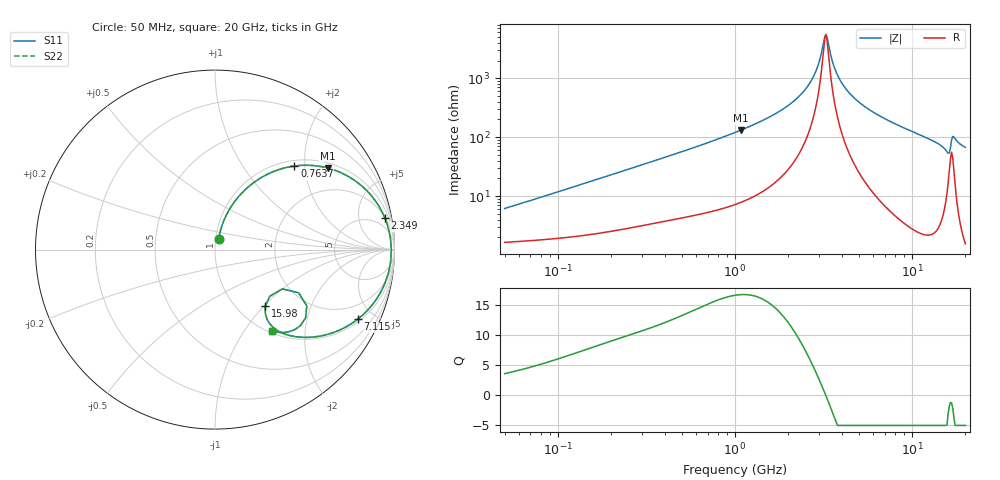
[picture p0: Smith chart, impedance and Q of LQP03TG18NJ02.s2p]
!Murata Part Number: LQP03TG18NJ02
!These Parameters are Measured in Series Mode Connection
!  o--[Z]--o
!Port1  Port2
!  o-------o
!Freq. Start=50[MHz] Stop=20[GHz], 401[Steps]
# Hz S RI R 50
!Freq.(Hz) S11(Real) S11(Imag) S21(Real) S21(Imag) S12(Real) S12(Imag) S22(Real) S22(Imag)
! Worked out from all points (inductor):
!   401 points, 50 MHz to 20 GHz, reference 50 ohm
!   read as one part in series: L = 18.8 nH near 51.52 MHz
!   highest Q = 16.8 at 1.078 GHz (marker M1), where L = 19.4 nH
!   self-resonance near 3.217 GHz
!   S11 on the Smith chart (normalised r, x): 50 MHz: 1.03, +0.12; 763.7 MHz: 1.11, +1.77; 2.349 GHz: 2, +10; 7.115 GHz: 1.13, -4.04; 15.98 GHz: 1.33, -1.02; 20 GHz: 1.03, -1.35
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5e7  0.0196 0.0575  0.9804 -0.0575  0.9804 -0.0575  0.0196 0.0575
1.364002e8  0.0439 0.148  0.9561 -0.148  0.9561 -0.148  0.0439 0.148
3.721004e8  0.1716 0.3369  0.8284 -0.3369  0.8284 -0.3369  0.1716 0.3369
7.636728e8  0.4427 0.4658  0.5573 -0.4658  0.5573 -0.4658  0.4427 0.4658
1e9  0.5861 0.4634  0.4139 -0.4634  0.4139 -0.4634  0.5861 0.4634
1.077769e9  0.6269 0.4547  0.3731 -0.4547  0.3731 -0.4547  0.6269 0.4547
1.714689e9  0.8516 0.3223  0.1484 -0.3223  0.1484 -0.3223  0.8516 0.3223
2.348516e9  0.9468 0.1751  0.0532 -0.1751  0.0532 -0.1751  0.9468 0.1751
2.728004e9  0.9713 0.0964  0.0287 -0.0964  0.0287 -0.0964  0.9713 0.0964
3.265178e9  0.9823 -0.0014  0.0177 0.0014  0.0177 0.0014  0.9823 -0.0014
3.680849e9  0.9784 -0.0671  0.0216 0.0671  0.0216 0.0671  0.9784 -0.0671
4.212059e9  0.9632 -0.1402  0.0368 0.1402  0.0368 0.1402  0.9632 -0.1402
5.194772e9  0.9165 -0.249  0.0835 0.249  0.0835 0.249  0.9165 -0.249
7.114996e9  0.7954 -0.3876  0.2046 0.3876  0.2046 0.3876  0.7954 -0.3876
7.442007e9  0.7736 -0.4037  0.2264 0.4037  0.2264 0.4037  0.7736 -0.4037
1.295331e10  0.4407 -0.4839  0.5593 0.4839  0.5593 0.4839  0.4407 -0.4839
1.482269e10  0.3343 -0.4417  0.6657 0.4417  0.6657 0.4417  0.3343 -0.4417
1.597544e10  0.28 -0.3153  0.72 0.3153  0.72 0.3153  0.28 -0.3153
1.646126e10  0.375 -0.2189  0.625 0.2189  0.625 0.2189  0.375 -0.2189
1.721783e10  0.5046 -0.3804  0.4954 0.3804  0.4954 0.3804  0.5046 -0.3804
1.800918e10  0.4238 -0.4543  0.5762 0.4543  0.5762 0.4543  0.4238 -0.4543
2e10  0.3157 -0.4534  0.6843 0.4534  0.6843 0.4534  0.3157 -0.4534
